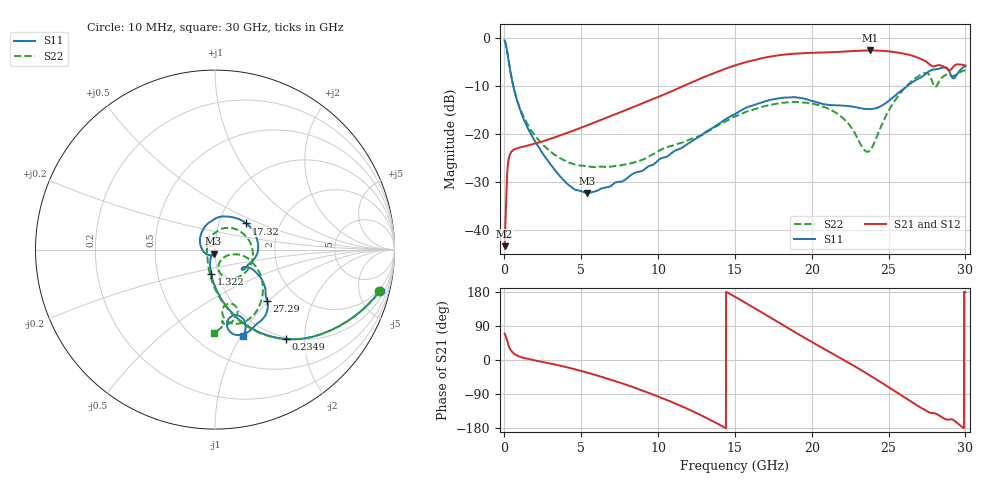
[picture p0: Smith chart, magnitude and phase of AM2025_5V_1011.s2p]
!Keysight Technologies,N5245B,MY58422270,A.16.20.02
!Date: Tuesday, July 14, 2026 01:09:04
!Correction: S11(C  2-Port  )
!S21(C  2-Port  )
!S12(C  2-Port  )
!S22(C  2-Port  )
!S2P File: Measurements: S11, S21, S12, S22:
# Hz S  dB  R 50
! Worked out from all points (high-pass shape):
!   3201 points, 10 MHz to 30 GHz, reference 50 ohm
!   highest |S21| = -2.56 dB at 23.82 GHz (marker M1); lowest = -43.4 dB at 10 MHz (marker M2)
!   |S21| within 3 dB of the highest: 15.12 GHz to 27.71 GHz (12.59 GHz wide, 58.8 % of centre); 29.35 GHz to 29.84 GHz (488.6 MHz wide, 1.65 % of centre)
!   lowest |S11| = -32.3 dB at 5.371 GHz (marker M3), VSWR 1.05, Z = 49.2 - j2.27 ohm
!   |S11| at or under -10 dB: 575.1 MHz to 26.21 GHz (25.63 GHz wide, 191 % of centre)
!   |S22| runs from -26.9 to -0.5 dB; largest |S21 - S12| = 0.0095
!   S11 on the Smith chart (normalised r, x): 10 MHz: 1.75, -7.78; 234.9 MHz: 0.97, -1.63; 1.322 GHz: 0.92, -0.25; 17.32 GHz: 1.35, +0.42; 27.29 GHz: 1.42, -0.98; 30 GHz: 0.78, -1.03
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1e7  -0.47 -14.0  -43.35 69.6  -36.09 87.0  -0.50 -14.3
2.34925e8  -3.92 -51.5  -25.95 42.4  -25.94 42.6  -3.94 -51.8
5.629406e8  -9.83 -78.6  -23.34 18.6  -23.37 18.9  -9.75 -79.1
1.322062e9  -17.38 -99.3  -22.53 4.8  -22.54 4.8  -16.87 -101.0
3.505709e9  -28.40 -118.7  -20.39 -13.9  -20.40 -13.9  -24.79 -136.5
5.014581e9  -31.91 -111.3  -18.62 -29.1  -18.62 -29.1  -26.56 -159.1
5.370712e9  -32.26 -108.5  -18.18 -33.1  -18.18 -33.0  -26.71 -164.9
1.000979e10  -25.43 -149.4  -12.23 -96.6  -12.21 -96.7  -23.56 128.0
1.274638e10  -20.36 150.8  -8.43 -144.8  -8.42 -144.8  -20.35 86.8
1.5005e10  -15.82 96.3  -5.69 166.8  -5.68 166.8  -16.31 51.9
1.616711e10  -14.02 67.1  -4.61 139.7  -4.61 139.7  -14.91 30.3
1.731985e10  -12.86 39.9  -3.82 111.9  -3.81 111.8  -13.90 8.5
1.863192e10  -12.33 10.2  -3.30 80.0  -3.30 79.9  -13.33 -16.9
2.000958e10  -13.07 -14.8  -3.05 47.4  -3.05 47.3  -13.63 -41.8
2.203391e10  -14.06 -31.8  -2.80 1.3  -2.81 1.2  -16.69 -75.2
2.382393e10  -14.80 -34.3  -2.56 -41.7  -2.56 -41.8  -23.26 -34.3
2.500479e10  -13.08 -27.5  -2.74 -71.9  -2.74 -71.9  -15.13 -13.5
2.609193e10  -10.28 -32.3  -3.27 -99.9  -3.28 -99.9  -10.24 -32.2
2.729153e10  -7.76 -44.6  -4.60 -130.5  -4.59 -130.5  -7.32 -63.6
2.805065e10  -6.50 -59.4  -5.80 -141.2  -5.78 -141.3  -10.15 -75.9
2.900658e10  -7.32 -81.0  -6.63 -156.7  -6.62 -156.9  -7.70 -83.9
3e10  -5.86 -72.0  -5.69 178.4  -5.68 178.3  -6.69 -90.8
